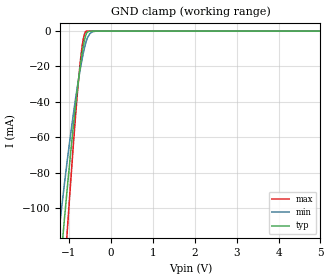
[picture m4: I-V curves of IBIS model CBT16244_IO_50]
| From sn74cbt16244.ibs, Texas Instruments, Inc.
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[Model]   CBT16244_IO_50
Model_type  Terminator
| variable   typ   min   max
C_comp   3.42pF   2.66pF   6.44pF
| C_tri-state   3.42pF   2.66pF   6.44pF
[Temperature Range]   40   100   -40
| Ambient temperature   25   85   -40
[Voltage range]   5   4.5   5.5
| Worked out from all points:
|   GND clamp passes 1 mA (typ) near -0.57 V on its own axis
[GND Clamp]
| CBT16244_IO_50
|   Voltage   I(typ)   I(min)   I(max)
-5V       -3.536A    -3.721A    -3.048A
-1.245V   -144.4mA   -115.7mA   -188.8mA
-1.18V    -126.4mA   -101.7mA   -164.4mA
-1.105V   -106.2mA   -86.31mA   -137mA
-1.03V    -86.88mA   -71.71mA   -110.4mA
-840mV    -42.12mA   -38.26mA   -48.02mA
-705mV    -15.97mA   -18.52mA   -12.62mA
-630mV    -5.474mA   -9.802mA   -1.886mA
-580mV    -1.347mA   -5.382mA   -55.45uA
-505mV    -73.79uA   -1.647mA   -2.79uA
-360mV    -723.9nA   -45.84uA   -8.648nA
5V        70.03pA    3.041nA    31.56pA
